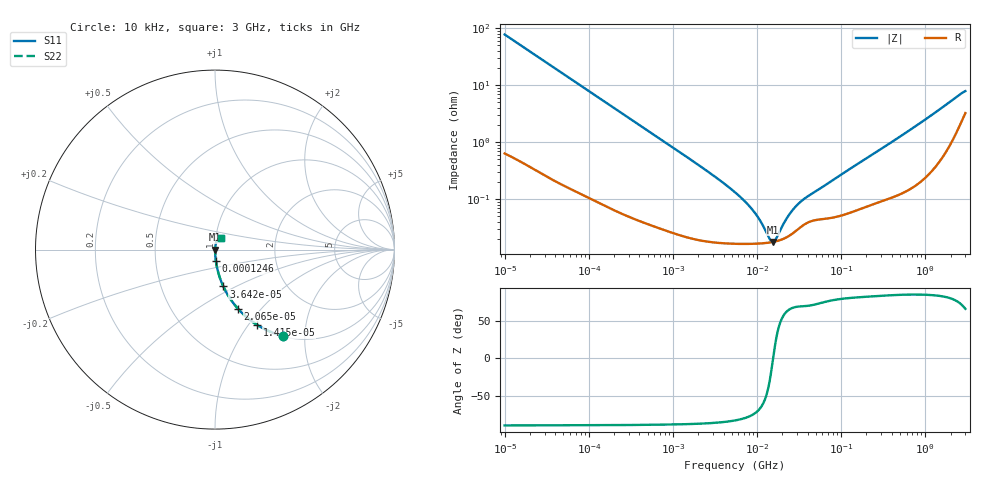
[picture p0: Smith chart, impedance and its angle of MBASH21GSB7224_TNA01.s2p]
! MBASH21GSB7224_TNA01  S-PARAMETER MODEL  ( Standard Model )
! Model Generated by TAIYO YUDEN Corporation (http://www.ty-top.com)
! Version 1.0
! TAIYO YUDEN Control No. 220601
! Copyright(c) 2013 TAIYO YUDEN CO.,LTD. All Rights Reserved.
! Product Description (link to TY-COMPAS)
! https://ds.yuden.co.jp/TYCOMPAS/or/detail?pn=MBASH21GSB7224KTNA01&u=M
! Products Name : Multilayer Ceramic Capacitors
! Characteristics :
!  Capacitance : 0.22 [uF] , Rated Voltage : 100 [V] , TCC : X7R
!  Case Size : 2.0 x 1.25 / 0.079 x 0.049 [mm/inch] , Thickness : 1.25 / 0.049 [mm/inch]
!  (Conditions: Temperature = 25 [degC] , DC Bias Voltage = 0 [V])
! External Node Assignments :
!  1  o---| |---o  2
! GND o---------o GND
! Frequency Range : 10kHz  -  3GHz  [ 401 STEP ]
# MHZ S RI R 50
! Freq[MHz].  S11 Real  S11 Imag  S21 Real  S21 Imag  S12 Real  S12 Imag  S22 Real  S22 Imag
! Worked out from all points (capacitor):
!   401 points, 10 kHz to 3 GHz, reference 50 ohm
!   read as one part in series: C = 204 nF near 10.65 kHz
!   lowest |Z| = 17.6 mohm at 15.5 MHz (marker M1)
!   series resonance near 15.55 MHz, so ESL is about 510 pH
!   S11 on the Smith chart (normalised r, x): 10 kHz: 1.01, -1.56; 14.15 kHz: 1.01, -1.10; 20.65 kHz: 1.01, -0.76; 36.42 kHz: 1.00, -0.43; 124.6 kHz: 1.00, -0.13; 3 GHz: 1.06, +0.14
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0.01  0.3789 -0.4811  0.6211 0.4811  0.6211 0.4811  0.3789 -0.4811
0.014146  0.2356 -0.42  0.7644 0.42  0.7644 0.42  0.2356 -0.42
0.020651  0.128 -0.3294  0.872 0.3294  0.872 0.3294  0.128 -0.3294
0.036425  0.0464 -0.2052  0.9536 0.2052  0.9536 0.2052  0.0464 -0.2052
0.082683  0.0102 -0.0944  0.9898 0.0944  0.9898 0.0944  0.0102 -0.0944
0.124573  0.0049 -0.0632  0.9951 0.0632  0.9951 0.0632  0.0049 -0.0632
0.683653  0.000444 -0.0117  0.9996 0.0117  0.9996 0.0117  0.000444 -0.0117
2.652321  0.000186 -0.00297  0.9998 0.00297  0.9998 0.00297  0.000186 -0.00297
5.477226  0.000165 -0.0013  0.9998 0.0013  0.9998 0.0013  0.000165 -0.0013
7.274378  0.000163 -0.000877  0.9998 0.000877  0.9998 0.000877  0.000163 -0.000877
9.070798  0.000164 -0.000595  0.9998 0.000595  0.9998 0.000595  0.000164 -0.000595
10.95979  0.000166 -0.000377  0.9998 0.000377  0.9998 0.000377  0.000166 -0.000377
14.10408  0.000172 -0.000104  0.9998 0.000104  0.9998 0.000104  0.000172 -0.000104
15.50326  0.000176 -3.34e-06  0.9998 3.34e-06  0.9998 3.34e-06  0.000176 -3.34e-06
17.04125  0.000182 9.73e-05  0.9998 -9.73e-05  0.9998 -9.73e-05  0.000182 9.73e-05
21.93027  0.000209 0.000373  0.9998 -0.000373  0.9998 -0.000373  0.000209 0.000373
26.49725  0.000249 0.000588  0.9998 -0.000588  0.9998 -0.000588  0.000249 0.000588
34.09912  0.000332 0.000872  0.9997 -0.000872  0.9997 -0.000872  0.000332 0.000872
45.28751  0.000414 0.00118  0.9996 -0.00118  0.9996 -0.00118  0.000414 0.00118
374.4521  0.0011 0.00935  0.9989 -0.00935  0.9989 -0.00935  0.0011 0.00935
2482.93  0.0211 0.0614  0.9789 -0.0614  0.9789 -0.0614  0.0211 0.0614
3000  0.036 0.0672  0.964 -0.0672  0.964 -0.0672  0.036 0.0672
